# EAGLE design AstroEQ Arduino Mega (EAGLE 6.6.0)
REVISION: V4.8
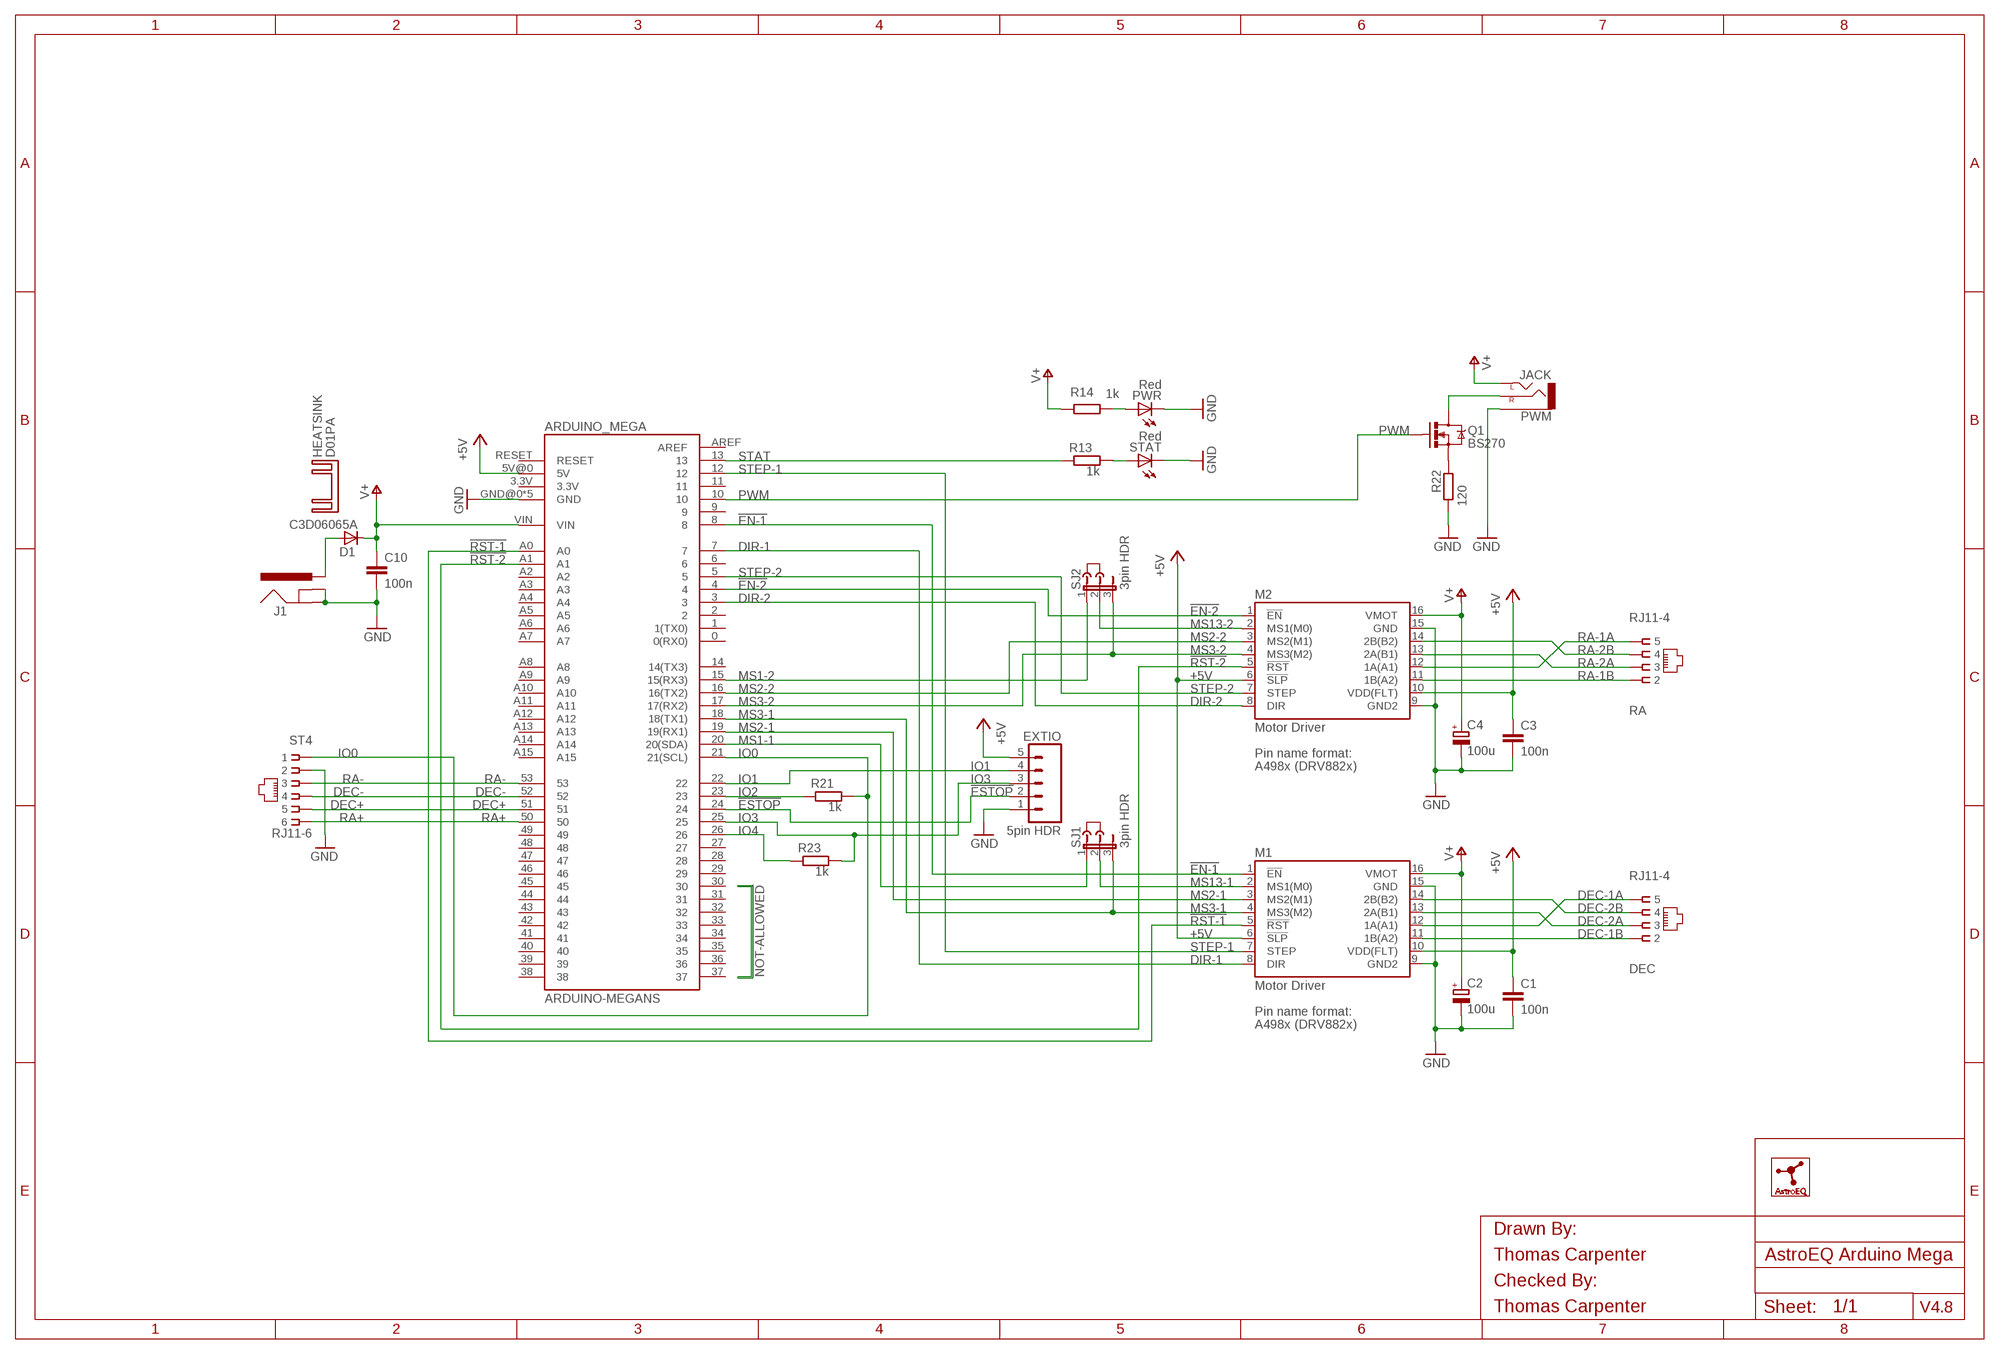
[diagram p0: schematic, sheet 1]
FRAME1 (A3L-LOC): CHECKED_BY: Thomas Carpenter; DRAWN_BY: Thomas Carpenter

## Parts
ARDUINO_MEGA  ARDUINO-MEGANS  [ARDUINO_MEGA_NS]
C1  100n  C-EU025-024X044  [C025-024X044]
C2  100u  CPOL-EUE2.5-7  [E2,5-7]
C3  100n  C-EU025-024X044  [C025-024X044]
C4  100u  CPOL-EUE2.5-7  [E2,5-7]
C10  100n  C-EU025-024X044  [C025-024X044]
D1  C3D06065A  MUR820VERT  [TO220ACS]
DEC  RJ11-4  [RJ11-NO_SHIELD-4]
EXTIO  5pin HDR  M05PTH  [1X05]
HEATSINK  D01PA  [D01PA]
J1  POWER_JACKPTH  [POWER_JACK_PTH]
J2  DNI  JUMPER  [JUMP]
J3  DNI  JUMPER  [JUMP]
LOGO1  ASTROEQ8MM  [ASTROEQ]
M1  Motor Driver  A4983CARRIER  [DIP16-W]
M2  Motor Driver  A4983CARRIER  [DIP16-W]
PWM  JACK  AUDIO-JACKVERT  [AUDIO-JACK-3.5MM-VERT]
PWR  Red  LED3MM  [LED3MM]
Q1  BS270  MOSFET-NCHANNELPTH  [TO-92]
R13  1k  R-EU_0204/5  [0204/5]
R14  1k  R-EU_0204/7  [0204/7]
R21  1k  R-EU_0204/7  [0204/7]
R22  120  R-EU_0204/7  [0204/7]
R23  1k  R-EU_0204/7  [0204/7]
RA  RJ11-4  [RJ11-NO_SHIELD-4]
SJ1  3pin HDR  JP2E  [JP2]
SJ2  3pin HDR  JP2E  [JP2]
ST4  RJ11-6  RJ11-2L-B  [RJ11-NO_SHIELD]
STAT  Red  LED3MM  [LED3MM]

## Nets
!EN-1: ARDUINO_MEGA.8 M1.1(!EN)
!EN-2: ARDUINO_MEGA.4 M2.1(!EN)
!ESTOP: ARDUINO_MEGA.24 EXTIO.2
!RST-1: ARDUINO_MEGA.A0 M1.5(!RST)
!RST-2: ARDUINO_MEGA.A1 M2.5(!RST)
+5V: ARDUINO_MEGA.5V@0(5V) C1.1 C3.1 EXTIO.5 M1.6(!SLP) M1.10(VDD(FLT)) M2.6(!SLP) M2.10(VDD(FLT))
DEC+: ARDUINO_MEGA.51 ST4.5
DEC-: ARDUINO_MEGA.52 ST4.4
DEC-1A: DEC.5 M1.12(1A(A1))
DEC-1B: DEC.2 M1.11(1B(A2))
DEC-2A: DEC.3 M1.13(2A(B1))
DEC-2B: DEC.4 M1.14(2B(B2))
DIR-1: ARDUINO_MEGA.7 M1.8(DIR)
DIR-2: ARDUINO_MEGA.3 M2.8(DIR)
GND: ARDUINO_MEGA.GND@0(GND) ARDUINO_MEGA.GND@1(GND) ARDUINO_MEGA.GND@2(GND) ARDUINO_MEGA.GND@3(GND) ARDUINO_MEGA.GND@4(GND) C1.2 C2.- C3.2 C4.- C10.2 EXTIO.1 J1.GND J1.GNDBREAK M1.9(GND2) M1.15(GND) M2.9(GND2) M2.15(GND) PWM.1(SLEEVE) PWR.K(C) R22.1 ST4.2 STAT.K(C)
IO0: ARDUINO_MEGA.21(21(SCL)) R21.2 ST4.1
IO1: ARDUINO_MEGA.22 EXTIO.4
IO2: ARDUINO_MEGA.23 R21.1
IO3: ARDUINO_MEGA.25 EXTIO.3 R23.2
IO4: ARDUINO_MEGA.26 R23.1
MS1-1: ARDUINO_MEGA.20(20(SDA)) SJ1.1
MS1-2: ARDUINO_MEGA.15(15(RX3)) SJ2.1
MS2-1: ARDUINO_MEGA.19(19(RX1)) M1.3(MS2(M1))
MS2-2: ARDUINO_MEGA.16(16(TX2)) M2.3(MS2(M1))
MS3-1: ARDUINO_MEGA.18(18(TX1)) M1.4(MS3(M2)) SJ1.3
MS3-2: ARDUINO_MEGA.17(17(RX2)) M2.4(MS3(M2)) SJ2.3
MS13-1: M1.2(MS1(M0)) SJ1.2
MS13-2: M2.2(MS1(M0)) SJ2.2
PWM: ARDUINO_MEGA.10 Q1.2(G)
PWM-ILIM: Q1.3(S) R22.2
PWM-OUT: PWM.3(RIGHT) Q1.1(D)
PWRLED: PWR.A R14.2
RA+: ARDUINO_MEGA.50 ST4.6
RA-: ARDUINO_MEGA.53 ST4.3
RA-1A: M2.12(1A(A1)) RA.5
RA-1B: M2.11(1B(A2)) RA.2
RA-2A: M2.13(2A(B1)) RA.3
RA-2B: M2.14(2B(B2)) RA.4
STAT: ARDUINO_MEGA.13 R13.1
STATLED: R13.2 STAT.A
STEP-1: ARDUINO_MEGA.12 M1.7(STEP)
STEP-2: ARDUINO_MEGA.5 M2.7(STEP)
V+: ARDUINO_MEGA.VIN C2.+ C4.+ C10.1 D1.C M1.16(VMOT) M2.16(VMOT) PWM.2(LEFT) R14.1
VIN: D1.A J1.PWR
Unconnected: ARDUINO_MEGA.0(0(RX0)) ARDUINO_MEGA.1(1(TX0)) ARDUINO_MEGA.2 ARDUINO_MEGA.3.3V ARDUINO_MEGA.6 ARDUINO_MEGA.9 ARDUINO_MEGA.11 ARDUINO_MEGA.14(14(TX3)) ARDUINO_MEGA.27 ARDUINO_MEGA.28 ARDUINO_MEGA.29 ARDUINO_MEGA.30 ARDUINO_MEGA.31 ARDUINO_MEGA.32 ARDUINO_MEGA.33 ARDUINO_MEGA.34 ARDUINO_MEGA.35 ARDUINO_MEGA.36 ARDUINO_MEGA.37 ARDUINO_MEGA.38 ARDUINO_MEGA.39 ARDUINO_MEGA.40 ARDUINO_MEGA.41 ARDUINO_MEGA.42 ARDUINO_MEGA.43 ARDUINO_MEGA.44 ARDUINO_MEGA.45 ARDUINO_MEGA.46 ARDUINO_MEGA.47 ARDUINO_MEGA.48 ARDUINO_MEGA.49 ARDUINO_MEGA.A2 ARDUINO_MEGA.A3 ARDUINO_MEGA.A4 ARDUINO_MEGA.A5 ARDUINO_MEGA.A6 ARDUINO_MEGA.A7 ARDUINO_MEGA.A8 ARDUINO_MEGA.A9 ARDUINO_MEGA.A10 ARDUINO_MEGA.A11 ARDUINO_MEGA.A12 ARDUINO_MEGA.A13 ARDUINO_MEGA.A14 ARDUINO_MEGA.A15 ARDUINO_MEGA.AREF ARDUINO_MEGA.RESET

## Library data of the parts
ARDUINO_MEGA = SparkFun:ARDUINO-MEGA: Arduino Mega footprint connections
C1 C3 C10 = resistor:C-EU: CAPACITOR, European symbol; MF: AVX; MPN: SR205C104KAR; OC_FARNELL: 1100367
C2 C4 = resistor:CPOL-EU: POLARIZED CAPACITOR, European symbol; MF: MULTICOMP; MPN: MCGPR25V107M6.3X11; OC_FARNELL: 9451188
D1 = diode:MUR820: DIODE; MF: CREE; MPN: C3D06065A; OC_FARNELL: 1864928
DEC RA = con-tycoelectronics:RJ11-4; MF: MOLEX; MPN: 95501-2641; OC_FARNELL: 1560166
EXTIO = SparkFun:M05: Header 5 Standard 5-pin 0.1" header. Use with straight break away headers (SKU : PRT-00116), right angle break away headers (PRT-00553), swiss pins (PRT-00743), machine pins (PRT-00117), and female headers (PRT-00115). Molex polarized connector foot print use with SKU : PRT-08230 with associated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; OC_FARNELL: unknown
HEATSINK = heatsink:D01PA: HEATSINK
J1 = SparkFun:POWER_JACK: Power Jack This is the standard 5.5mm barrel jack for power. The PTH is the most common, proven, reliable, footprint. All others are experimental. The Slot footprint only works if the mill layer is transmitted to the PCB fab house so be warned. Spark Fun Electronics SKU : PRT-00119. Mating wall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; MF: MULTICOMP; MPN: MJ-179PH; OC_FARNELL: 1737246
J2 J3 = jumper:JUMPER: JUMPER header; MF: 3M; MPN: 969102-0000-DA; OC_FARNELL: 2579814
LOGO1 = CompanyLogos:ASTROEQ
M1 M2 = A4983Carrier:A4983CARRIER; MF: SAMTEC; MPN: CES-116-01-T-S; OC_FARNELL: 1667522
PWM = SparkFun:AUDIO-JACK: 3.5mm Audio Jack Simple 3.5mm common PCB mount audio jack. SKU: PRT-08032; MANUFACTURER: LUMBERG; MF: CLIFF ELECTRONIC COMPONENTS; MPN: 1502 01; OC_FARNELL: 1243242
PWR STAT = led:LED: LED; MF: KINGBRIGHT; MPN: L-424HDT; OC_FARNELL: 1142499
Q1 = SparkFun:MOSFET-NCHANNEL; MF: FAIRCHILD SEMICONDUCTOR; MPN: BS270; OC_FARNELL: 1017689
R13 R14 R21 R23 = rcl:R-EU_: RESISTOR, European symbol; MF: MULTICOMP; MPN: MF12 1K; OC_FARNELL: 9342400
R22 = rcl:R-EU_: RESISTOR, European symbol; MF: MULTICOMP; MPN: MF12 120R; OC_FARNELL: 9342516
SJ1 SJ2 = jumper:JP2E: JUMPER; MF: HARWIN; MPN: M20-9990345.; OC_FARNELL: 1022248
ST4 = con-tycoelectronics:RJ11: CORCOM Modular RJ Jacks No Shield Source: www.tycoelectronics.com .. ENG_DS_1654001_1099_RJ_L_0507.pdf; MF: TYCO ELECTRONICS; MPN: RJ11-2L-B; OC_FARNELL: unknown; OC_NEWARK: 83F4463

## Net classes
1 power: width 0.61 mm, drill 0.711 mm, clearance 0.203 mm
2 gnd: width 0.305 mm, drill 0.711 mm, clearance 0.203 mm
3 usbvcc: width 0.508 mm, drill 0.711 mm, clearance 0.203 mm

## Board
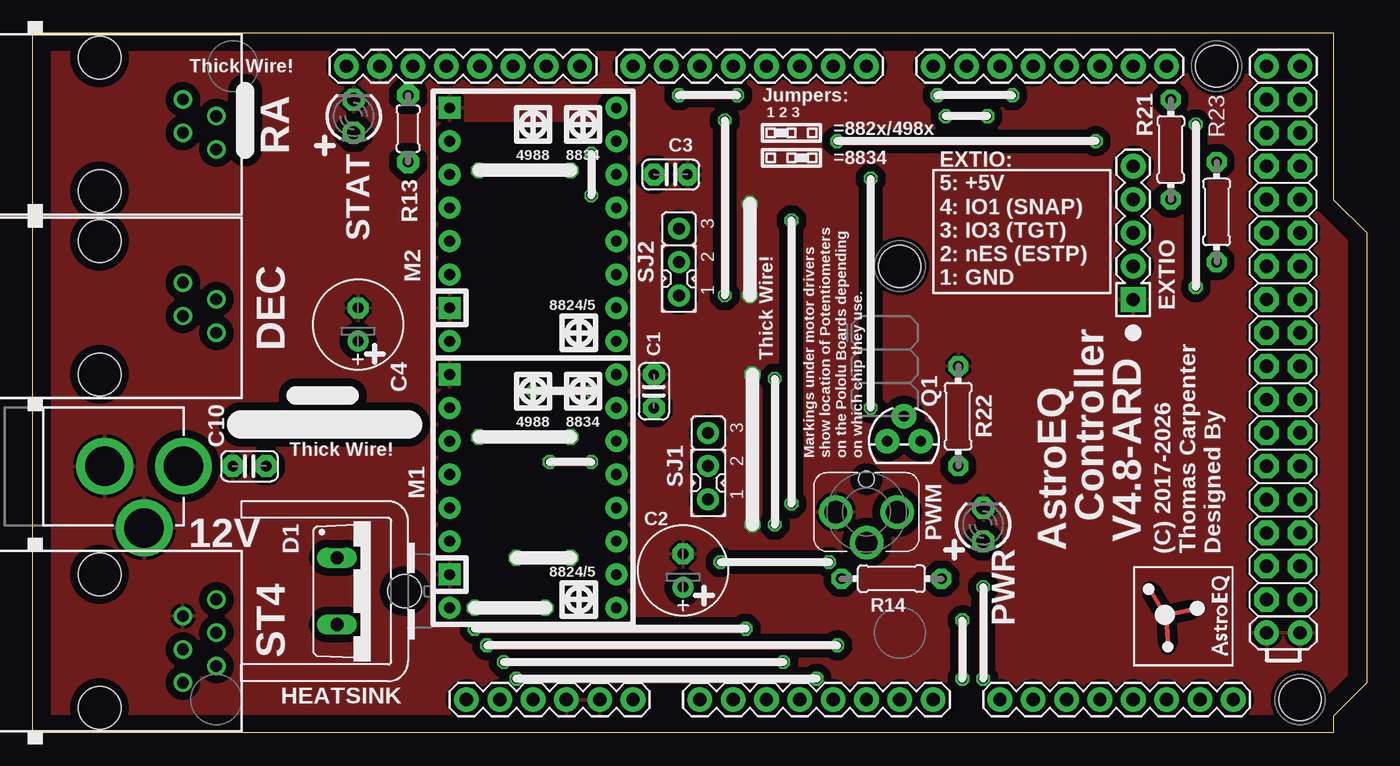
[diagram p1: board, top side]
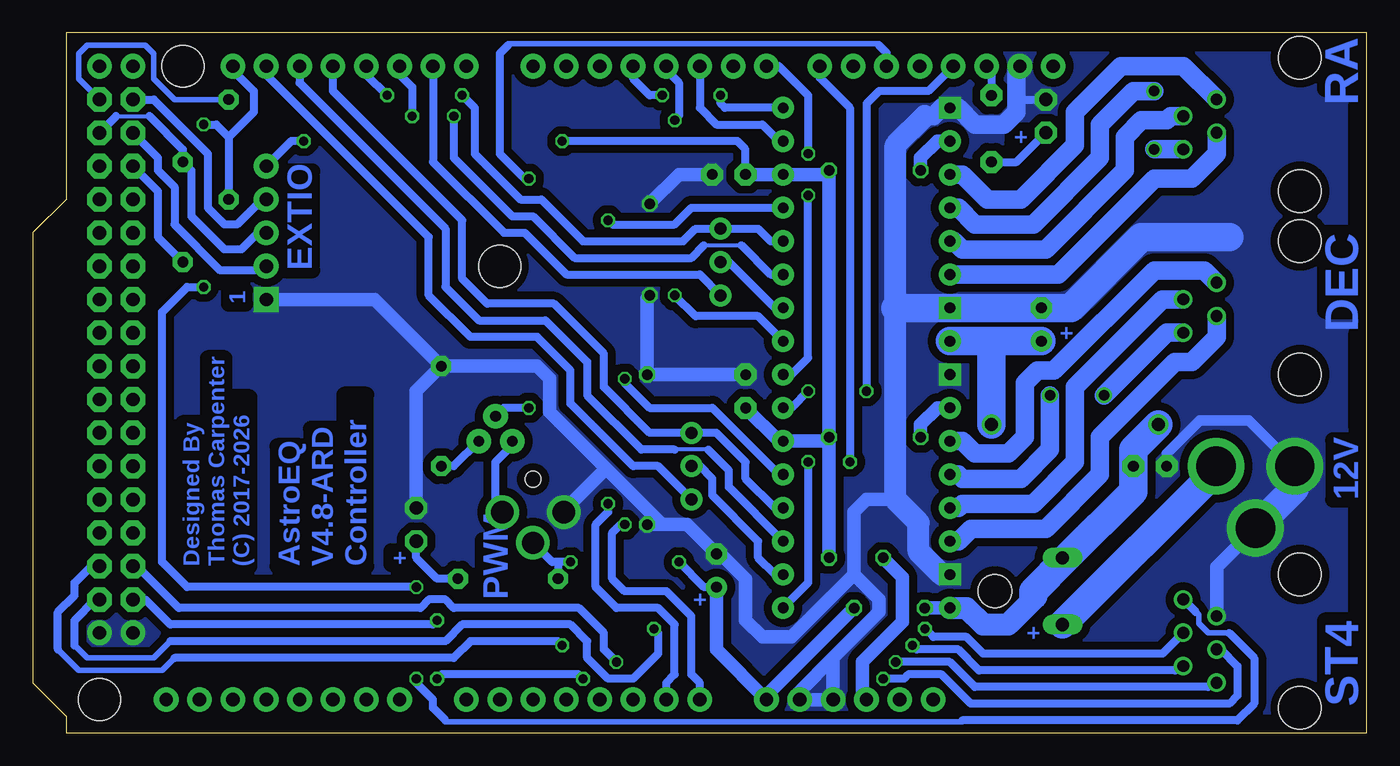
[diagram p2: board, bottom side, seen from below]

Size 101.6 x 53.34 mm. Coordinates in mm from the lower left corner, seen from the top.
Copper layers (1*16): Top 0.035mm / dielectric 1.5mm / Bottom 0.035mm
Design rules "default *": minimum track width 6mil, minimum drill 12mil, track to track 6mil, track to pad 6mil, pad to pad 6mil, via to via 6mil, smd to smd 0mil, copper to edge 12mil, drill to drill 10mil, minimum pad ring 10mil, minimum via ring 6mil, stop-mask expansion 2mil, vias tented up to drill 1mm, thermal gap 10mil
Holes 3.2 mm at 90.17,50.8 66.04,35.56 96.52,2.54
tRestrict: 8 lines
bRestrict: 10 lines

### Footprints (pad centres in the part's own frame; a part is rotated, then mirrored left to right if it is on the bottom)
ARDUINO_MEGA_NS = drill 1.016 pad 1.88: 0 63.5,50.8; 1 60.96,50.8; 2 58.42,50.8; 3 55.88,50.8; 3.3V 35.56,2.54; 4 53.34,50.8; 5 50.8,50.8; 5V@0 38.1,2.54; 5V@1 93.98,50.8; 5V@2 96.52,50.8; 6 48.26,50.8; 7 45.72,50.8; 8 41.656,50.8; 9 39.116,50.8; 10 36.576,50.8; 11 34.036,50.8; 12 31.496,50.8; 13 28.956,50.8; 14 68.58,50.8; 15 71.12,50.8; 16 73.66,50.8; 17 76.2,50.8; 18 78.74,50.8; 19 81.28,50.8; 20 83.82,50.8; 21 86.36,50.8; A0 50.8,2.54; A1 53.34,2.54; A2 55.88,2.54; A3 58.42,2.54; A4 60.96,2.54; A5 63.5,2.54; A6 66.04,2.54; A7 68.58,2.54; A8 73.66,2.54; A9 76.2,2.54; A10 78.74,2.54; A11 81.28,2.54; A12 83.82,2.54; A13 86.36,2.54; A14 88.9,2.54; A15 91.44,2.54; AREF 23.876,50.8; GND@0 40.64,2.54; GND@1 43.18,2.54; GND@2 93.98,7.62; GND@3 96.52,7.62; GND@4 26.416,50.8; RESET 33.02,2.54; VIN 45.72,2.54 | drill 1.016 pad 1.88 octagon: 22 93.98,48.26; 23 96.52,48.26; 24 93.98,45.72; 25 96.52,45.72; 26 93.98,43.18; 27 96.52,43.18; 28 93.98,40.64; 29 96.52,40.64; 30 93.98,38.1; 31 96.52,38.1; 32 93.98,35.56; 33 96.52,35.56; 34 93.98,33.02; 35 96.52,33.02; 36 93.98,30.48; 37 96.52,30.48; 38 93.98,27.94; 39 96.52,27.94; 40 93.98,25.4; 41 96.52,25.4; 42 93.98,22.86; 43 96.52,22.86; 44 93.98,20.32; 45 96.52,20.32; 46 93.98,17.78; 47 96.52,17.78; 48 93.98,15.24; 49 96.52,15.24; 50 93.98,12.7; 51 96.52,12.7; 52 93.98,10.16; 53 96.52,10.16
C025-024X044 = drill 0.813 pad 1.676 octagon: 1 -1.27,0; 2 1.27,0
E2,5-7 = drill 0.813 pad 1.6: + -1.27,0 | drill 0.813 pad 1.6 octagon: - 1.27,0
TO220ACS = drill 1.016 long: A 2.54,-2.54; C -2.54,-2.54
RJ11-NO_SHIELD-4 = drill 0.9 pad 1.4: 2 -1.905,6.35; 3 -0.635,8.89; 4 0.635,6.35; 5 1.905,8.89 | hole 3.251: -5.08,0; 5.08,0
1X05 = drill 1.016 pad 1.88 square: 1 -5.08,0 | drill 1.016 pad 1.88: 2 -2.54,0; 3 0,0; 4 2.54,0; 5 5.08,0
D01PA = hole 2.54: 0,-1.016
POWER_JACK_PTH = drill 2.997 pad 4.318: GND 0,7.7; GNDBREAK 4.7,10.7; PWR 0,13.7
DIP16-W = drill 0.813 pad 1.676: 1 -8.89,-6.35; 2 -6.35,-6.35; 3 -3.81,-6.35; 4 -1.27,-6.35; 5 1.27,-6.35; 6 3.81,-6.35; 7 6.35,-6.35; 8 8.89,-6.35; 10 6.35,6.35; 11 3.81,6.35; 12 1.27,6.35; 13 -1.27,6.35; 14 -3.81,6.35; 16 -8.89,6.35 | drill 0.813 pad 1.676 square: 9 8.89,6.35; 15 -6.35,6.35
AUDIO-JACK-3.5MM-VERT = drill 1.7: 1 2.35,0; 2 0,2.35; 3 -2.35,0 | hole 1.2: 0,-2.5
LED3MM = drill 1 pad 1.676 octagon: A -1.27,0; K 1.27,0
TO-92 = drill 0.813 pad 1.88: 1 -1.27,0; 2 0,1.905; 3 1.27,0
0204/5 = drill 0.813 pad 1.676 octagon: 1 -2.54,0; 2 2.54,0
0204/7 = drill 0.813 pad 1.524 octagon: 1 -3.81,0; 2 3.81,0
JP2 = drill 0.914 pad 1.676: 1 -2.54,0; 2 0,0; 3 2.54,0
RJ11-NO_SHIELD = drill 0.9 pad 1.4: 1 -3.175,8.89; 2 -1.905,6.35; 3 -0.635,8.89; 4 0.635,6.35; 5 1.905,8.89; 6 3.175,6.35 | hole 3.251: -5.08,0; 5.08,0

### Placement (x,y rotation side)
ARDUINO_MEGA  0,0 0 top
C1  47.31,26.02 90 top
C2  49.53,12.37 90 top
C3  48.59,42.55 0 top
C4  24.77,31.11 90 top
C10  16.5,20.32 180 top
D1  25.72,10.79 270 top
DEC  5.08,32.4 270 top
EXTIO  83.82,38.1 90 top
HEATSINK  27.3,10.79 90 top
J1  -2.22,20.31 270 top
J2  49.21,34.61 180 top
J3  51.44,19.05 180 top
LOGO1  91.44,5.08 90 top
M1  38.1,18.41 90 top
M2  38.1,38.73 90 top
PWM  63.5,16.83 180 top
PWR  72.39,15.88 90 top
Q1  66.36,22.23 0 top
R13  28.59,46.04 270 top
R14  65.41,11.75 0 top
R21  86.68,44.45 270 top
R22  70.48,24.13 270 top
R23  90.17,39.69 90 top
RA  5.08,46.37 270 top
SJ1  51.44,20.32 90 top
SJ2  49.21,35.88 90 top
ST4  5.08,7 270 top
STAT  24.45,46.99 90 top

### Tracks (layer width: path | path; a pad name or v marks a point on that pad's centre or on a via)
!EN-1  (via drill 0.7)
  Top 0.61: v39.37,20.64 v42.55,20.64
  Bottom 0.61: ARDUINO_MEGA.8 41.66,49.91 39.37,47.62 v39.37,20.64 | v42.55,20.64 42.55,11.43 M1.1
!EN-2  (via drill 0.7)
  Top 0.61: v52.7,33.34 v52.7,46.67
  Bottom 0.61: ARDUINO_MEGA.4 53.34,50.48 52.39,49.53 52.39,46.99 v52.7,46.67 | M2.1 46.35,31.75 51.12,31.75 v52.7,33.34
!ESTOP
  Bottom 0.61: ARDUINO_MEGA.24 92.08,43.81 92.08,42.86 90.81,41.59 90.81,38.73 87.31,35.24 84.14,35.24 EXTIO.2
!RST-1  (via drill 0.7)
  Top 0.61: v56.52,15.88 v56.52,26.99
  Bottom 0.61: ARDUINO_MEGA.A0 50.8,3.81 51.44,4.45 51.44,8.89 53.34,10.79 56.52,10.79 57.47,11.75 57.47,15.24 56.83,15.88 v56.52,15.88 | v56.52,26.99 56.52,26.67 54.61,24.77 49.85,24.77 44.77,19.68 M1.5
!RST-2  (via drill 0.7)
  Top 0.61: v57.78,17.46 v57.78,39.05
  Bottom 0.61: ARDUINO_MEGA.A1 53.34,3.81 52.7,4.45 52.7,8.26 53.98,9.53 57.15,9.53 58.74,11.11 58.74,15.88 57.78,16.83 v57.78,17.46 | v57.78,39.05 57.47,38.73 52.7,38.73 51.44,40.01 M2.5
+5V  (via drill 0.7, 0.8)
  Top 0.61: v61.28,45.09 v80.96,45.09
  Top 1.016: v33.97,22.54 v40.96,22.54 | v33.97,42.86 v40.96,42.86 | v36.83,13.34 v40.96,13.34
  Bottom 0.61: C3.1 47.32,44.46 47.94,45.09 v61.28,45.09 | v80.96,45.09 81.92,45.09 EXTIO.5
  Bottom 1.016: M1.10 32.7,24.77 33.97,23.5 v33.97,22.54 | 40.96,22.23 v40.96,22.54 40.96,42.55 | M2.10 32.7,45.09 33.97,43.81 v33.97,42.86 | v40.96,42.86 40.96,42.55 | 40.96,42.55 M2.6 C3.1 | 40.96,22.23 M1.6 44.78,22.23 C1.1 | v36.83,13.34 35.36,11.87 35.36,8.46 38.42,5.4 38.42,2.86 ARDUINO_MEGA.5V@0 | v40.96,13.34 40.96,22.23
DEC+  (via drill 0.7)
  Top 0.61: v34.61,6.67 v61.28,6.67
  Bottom 0.406: 90.81,5.71 91.76,4.76 98.11,4.76 99.69,6.35
  Bottom 0.61: ST4.5 14.29,5.08 14.61,4.76 29.53,4.76 31.11,6.35 34.29,6.35 v34.61,6.67 | v61.28,6.67 61.59,6.99 68.26,6.99 69.53,5.71 90.81,5.71 | 99.69,6.35 99.69,9.21 98.42,10.48 98.42,11.43 97.16,12.7 ARDUINO_MEGA.51
DEC-  (via drill 0.7)
  Top 0.61: v36.83,4.13 v59.69,4.13 | v70.8,4.13 v70.8,8.57
  Bottom 0.61: ST4.4 11.11,6.35 9.84,5.08 9.84,2.86 10.48,2.22 30.16,2.22 32.38,4.45 34.92,4.45 35.24,4.13 v36.83,4.13 | v59.69,4.13 60.01,4.45 70.48,4.45 v70.8,4.13 | v70.8,8.57 71.12,8.26 91.12,8.26 93.03,10.16 ARDUINO_MEGA.52
DEC-1A  (via drill 0.8)
  Top 1.422: v24.13,25.72 v20,25.72
  Bottom 1.422: v24.13,25.72 24.13,21.59 26.35,19.37 30.8,19.37 31.11,19.68 M1.12 | v20,25.72 15.23,30.49 DEC.5
DEC-1B
  Bottom 1.422: DEC.2 12.38,35.24 16.19,35.24 23.81,27.62 25.08,27.62 26.04,26.67 26.04,22.54 27.3,21.27 29.84,21.27 30.8,22.23 M1.11
DEC-2A
  Bottom 1.422: M1.13 31.11,17.14 30.8,17.46 25.4,17.46 22.23,20.64 22.23,26.35 15.55,33.03 DEC.3
DEC-2B
  Bottom 1.422: DEC.4 11.43,30.16 13.34,28.26 14.61,28.26 20.32,22.54 20.32,19.68 24.45,15.56 30.16,15.56 31.11,14.61 M1.14
DIR-1  (via drill 0.7)
  Top 0.61: v42.55,40.96 v42.55,44.13
  Bottom 0.61: ARDUINO_MEGA.7 44.77,50.8 42.55,48.58 v42.55,44.13 | M1.8 43.81,27.3 42.55,28.57 v42.55,40.96
DIR-2  (via drill 0.7)
  Top 0.61: v49.21,48.58 v53.66,48.58
  Bottom 0.61: M2.8 48.9,47.62 49.21,47.94 v49.21,48.58 | v53.66,48.58 54.61,48.58 55.88,49.85 ARDUINO_MEGA.3
GND  (via drill 0.8)
  Top 1.016: v54.81,15.88 v54.81,27.3 | v54.61,33.34 v54.61,40.32
  Bottom 0.61: ST4.2 11.75,8.89 | 26.67,48.26 STAT.K
  Bottom 0.813: C10.2 15.23,21.28 12.7,23.81 8.98,23.81 J1.GND
  Bottom 1.016: 40.64,5.71 ARDUINO_MEGA.GND@0 ARDUINO_MEGA.GND@1 43.18,3.17 40.64,5.71 | 40.64,5.71 37.15,9.21 37.15,10.16 39.05,12.06 | 39.05,12.06 39.05,16.83 38.1,17.78 35.88,17.78 | 39.05,12.06 43.81,7.3 46.04,7.3 47.31,8.57 47.31,11.75 49.2,13.64 C2.- 51.76,15.88 53.66,15.88 | 53.66,15.88 57.94,20.16 | 57.94,20.16 62.23,24.45 62.23,26.99 63.18,27.94 R22.1 | R22.1 72.39,26.04 PWR.K | v54.61,40.32 52.39,42.55 C3.2 | v54.81,15.88 53.66,15.88 | v54.61,33.34 54.81,33.14 v54.81,27.3 47.31,27.3 | R22.1 75.56,33.02 EXTIO.1 | ST4.2 11.43,12.66 J1.GNDBREAK | PWM.1 61.15,16.95 57.94,20.16
  Bottom 1.422: 33.66,46.99 33.02,46.99 32.38,47.62 M2.9 31.11,47.62 29.84,46.35 27.62,46.35 26.67,47.31 26.67,48.26 26.67,50.55 ARDUINO_MEGA.GND@4
  Bottom 1.676: M1.15 32.38,12.06 34.13,13.81 34.13,16.03 35.88,17.78 35.88,32.38 35.88,44.77 33.66,46.99
  Bottom 2.184: J1.GND 5.48,18.61 J1.GNDBREAK | 10.48,37.78 17.14,37.78 22.54,32.38 M2.15 35.88,32.38
  pour Bottom (isolate 0.61, no thermals): -0.64,-0.64 102.87,-0.64 102.87,53.98 -0.64,53.98
  pour Top (isolate 0.61): -0.64,-0.64 102.87,-0.64 102.87,53.98 31.75,53.98 31.75,46.67 44.13,46.67 44.13,8.26 31.75,8.26 31.75,53.98 -0.64,53.98
IO0  (via drill 0.7)
  Top 0.61: v72.39,4.13 v72.39,11.11 | v88.58,33.97 v88.58,46.35
  Bottom 0.4: 13.02,9.22 13.02,9.21 12.8,8.99 12.8,8.36 12.06,7.62 10.48,7.62
  Bottom 0.406: 30.8,0.95 30.8,0.85 70.17,0.85 70.17,0.95
  Bottom 0.61: ARDUINO_MEGA.21 86.36,50.48 84.77,48.9 84.77,47.31 86.68,45.4 | 86.68,45.4 R21.2 | ST4.1 13.02,9.22 | 10.48,7.62 8.57,5.71 8.57,2.22 9.84,0.95 30.8,0.95 | 70.17,0.95 71.12,1.91 71.12,2.54 72.39,3.81 v72.39,4.13 | v72.39,11.11 89.85,11.11 91.76,13.02 91.76,32.07 89.85,33.97 v88.58,33.97 | v88.58,46.35 87.63,46.35 86.68,45.4
IO1
  Bottom 0.61: ARDUINO_MEGA.22 92.39,48.26 88.27,44.13 88.27,40.01 87,38.73 86.04,38.73 84.14,40.64 EXTIO.4
IO2
  Bottom 0.406: ARDUINO_MEGA.23 98.11,49.85 98.11,51.75 97.47,52.39 93.03,52.39 92.39,51.75 92.39,49.85 90.81,48.26 R21.1
IO3
  Bottom 0.3: 95.25,46.99 92.71,46.99
  Bottom 0.61: ARDUINO_MEGA.25 95.25,46.99 | 92.71,46.99 90.17,44.45 R23.2 89.53,42.86 89.53,39.37 87,36.83 85.72,36.83 84.45,38.1 EXTIO.3
IO4
  Bottom 0.61: ARDUINO_MEGA.26 92.08,41.27 92.08,37.78 R23.1
MS1-1
  Bottom 0.61: SJ1.1 53.98,20.32 55.88,20.32 60.64,25.08 60.64,27.62 63.18,30.16 68.26,30.16 71.44,33.34 71.44,37.78 83.82,50.16 ARDUINO_MEGA.20
MS1-2
  Bottom 0.61: ARDUINO_MEGA.15 71.12,43.5 65.72,38.1 64.14,38.1 60.96,34.92 50.8,34.92 SJ2.1
MS2-1
  Bottom 0.3: 50.16,21.59 52.7,21.59
  Bottom 0.61: M1.3 48.58,18.73 48.58,20 50.16,21.59 | 52.7,21.59 55.24,21.59 59.37,25.72 59.37,28.26 62.55,31.43 67.63,31.43 70.17,33.97 70.17,38.42 81.28,49.53 ARDUINO_MEGA.19
MS2-2  (via drill 0.7)
  Top 0.61: v72.71,46.99 v69.53,46.99
  Bottom 0.3: 50.48,37.15 47.62,37.15
  Bottom 0.61: ARDUINO_MEGA.16 73.66,50.16 72.71,49.21 v72.71,46.99 | v69.53,46.99 69.53,43.81 65.09,39.37 63.5,39.37 60.33,36.2 51.44,36.2 50.48,37.15 | 47.62,37.15 45.4,34.92 M2.3
MS3-1
  Bottom 0.61: M1.4 45.09,17.14 47.31,19.37 47.31,20.64 49.53,22.86 SJ1.3 54.61,22.86 58.1,26.35 58.1,28.89 61.91,32.7 66.99,32.7 68.9,34.61 68.9,39.05 78.74,48.9 ARDUINO_MEGA.18
MS3-2  (via drill 0.7)
  Top 0.61: v74.61,48.58 v68.9,48.58
  Bottom 0.61: ARDUINO_MEGA.17 76.2,50.16 v74.61,48.58 | v68.9,48.58 67.94,47.62 67.94,44.13 64.45,40.64 62.87,40.64 59.69,37.47 52.07,37.47 51.12,38.42 SJ2.3 46.35,38.42 45.4,37.47 M2.4
MS13-1
  Bottom 0.61: M1.2 45.09,12.06 46.35,13.34 46.35,14.61 49.85,18.1 49.85,19.37 50.8,20.32 SJ1.2
MS13-2
  Bottom 0.61: M2.2 45.09,32.38 48.58,35.88 SJ2.2
PWM  (via drill 0.7)
  Top 0.61: v63.82,42.23 v63.82,24.77
  Bottom 0.406: 37.15,52.39 37.15,52.49 65.41,52.49 65.41,52.39
  Bottom 0.61: ARDUINO_MEGA.10 36.58,51.82 37.15,52.39 | 65.41,52.39 66.04,51.75 66.04,44.13 64.14,42.23 v63.82,42.23 | v63.82,24.77 65.72,24.77 Q1.2
PWM-ILIM
  Bottom 0.61: Q1.3 69.53,20.32 R22.2
PWM-OUT
  Bottom 0.61: PWM.3 66.36,17.34 66.36,20.64 65.09,21.91 Q1.1
PWRLED
  Bottom 0.61: R14.2 70.8,11.75 72.39,13.34 PWR.A
RA+  (via drill 0.7)
  Top 0.61: v35.88,5.4 v57.15,5.4
  Bottom 0.61: ST4.6 11.75,3.81 12.06,3.49 29.84,3.49 31.75,5.4 v35.88,5.4 | v57.15,5.4 58.1,6.35 58.1,7.62 60.01,9.53 69.53,9.53 70.17,10.16 71.44,10.16 72.07,9.53 90.49,9.53 93.66,12.7 ARDUINO_MEGA.50
RA-  (via drill 0.7)
  Top 0.61: v33.66,7.94 v54.29,7.94
  Bottom 0.406: 91.12,6.99 92.39,5.71 97.47,5.71 98.42,6.67
  Bottom 0.61: ST4.3 15.56,6.03 29.21,6.03 30.48,7.3 33.02,7.3 v33.66,7.94 | v54.29,7.94 53.98,7.62 53.98,6.03 55.88,4.13 57.78,4.13 59.37,5.71 59.37,6.99 60.64,8.26 68.9,8.26 70.17,6.99 91.12,6.99 | 98.42,6.67 98.42,8.57 96.84,10.16 ARDUINO_MEGA.53
RA-1A  (via drill 0.8)
  Top 1.422: v16.19,48.9 v16.19,44.46
  Bottom 1.422: v16.19,44.46 RA.5 | v16.19,48.9 17.78,48.9 20.32,46.35 20.32,43.81 25.4,38.73 29.84,38.73 31.11,40.01 M2.12
RA-1B
  Bottom 1.422: RA.2 13.96,50.8 18.73,50.8 22.23,47.31 22.23,44.77 26.35,40.64 28.89,40.64 30.8,42.55 M2.11
RA-2A
  Bottom 1.422: RA.3 14.92,46.99 15.24,46.67 17.14,46.67 18.41,45.4 18.41,42.86 24.45,36.83 30.8,36.83 31.43,37.47 M2.13
RA-2B
  Bottom 1.422: M2.14 23.5,34.92 16.19,42.23 13.34,42.23 11.43,44.13 RA.4
STAT
  Bottom 0.61: ARDUINO_MEGA.13 28.59,50.43 R13.1
STATLED
  Bottom 0.61: R13.2 26.67,43.5 STAT.A
STEP-1  (via drill 0.7)
  Top 0.61: v38.1,26.04 v42.55,26.04
  Bottom 0.61: v38.1,26.04 38.1,47.94 37.15,48.9 33.4,48.9 ARDUINO_MEGA.12 | v42.55,26.04 43.81,24.77 M1.7
STEP-2
  Bottom 0.61: ARDUINO_MEGA.5 50.8,47.62 49.53,46.35 46.04,46.35 44.77,45.09 M2.7
V+  (via drill 0.7, 0.8, 1)
  Top 0.61: v52.39,13.02 v60.64,13.02
  Top 1.016: v33.66,9.53 v39.05,9.53
  Top 2.184: v15.88,23.5 v28.57,23.5
  Bottom 0.61: C2.+ 50.47,11.1 v52.39,13.02 | v60.64,13.02 61.59,13.02 | 61.59,13.02 R14.1 | 61.59,13.02 62.04,13.02 PWM.2
  Bottom 0.813: C10.1
  Bottom 1.016: v39.05,9.53 45.72,2.86 ARDUINO_MEGA.VIN 49.53,6.35 C2.+ | M1.16 v33.66,9.53
  Bottom 1.676: M1.16 30.48,9.53 29.21,8.26 27.3,8.26 25.4,10.16 25.4,10.48 | 22.86,13.34 D1.C
  Bottom 2.184: v15.88,23.5 17.78,21.59 C10.1 17.78,18.41 22.86,13.34 25.4,10.79 25.4,10.48 | v28.57,23.5 28.57,29.84 | 28.57,29.84 M2.16 | 28.57,29.84 C4.+
VIN
  Bottom 2.184: 11.16,20.27 11.27,20.16 | 11.27,20.16 D1.A | J1.PWR 11.42,20.31 11.27,20.16

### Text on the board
Bottom: RA | + | DEC | EXTIO | 1 | + | 12V | + | Controller | V4.8-ARD | AstroEQ | (C) 2017-2026 | Thomas Carpenter | Designed By | + | PWM | ST4 | +
tPlace: Thick Wire! | Jumpers: | 1 2 3 | =882x/498x | =8834 | Thick Wire! | Thick Wire! | Markings under motor drivers / show location of Potentiometers / on the Pololu Boards depending / on which chip they use.
tNames: EXTIO: / 5: +5V / 4: IO1 (SNAP) / 3: IO3 (TGT) / 2: nES (ESTP) / 1: GND | Controller | V4.8-ARD | AstroEQ | 12V | (C) 2017-2026 | Thomas Carpenter | Designed By
Reference: This board design is for Arduino Mega based AstroEQ controllers. | It is a 2 Layer board designed to be sent for manufacture. The AstroEQ-ARD-Gerber.zip file contains the required gerber files. | It can also be home etched as a 1 Layer board, using only the bottom, and making sure all white lines are connected with wires. | Make sure to show the ground plane. Type 'ratsnest' and press enter. | For printing the silkscreen to paper, you should only have TNames, TPlace and Dimension layers visible.

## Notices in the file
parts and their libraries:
SparkFun: Licensing: CC v3.0 Share-Alike You are welcome to use this library for commercial purposes.
